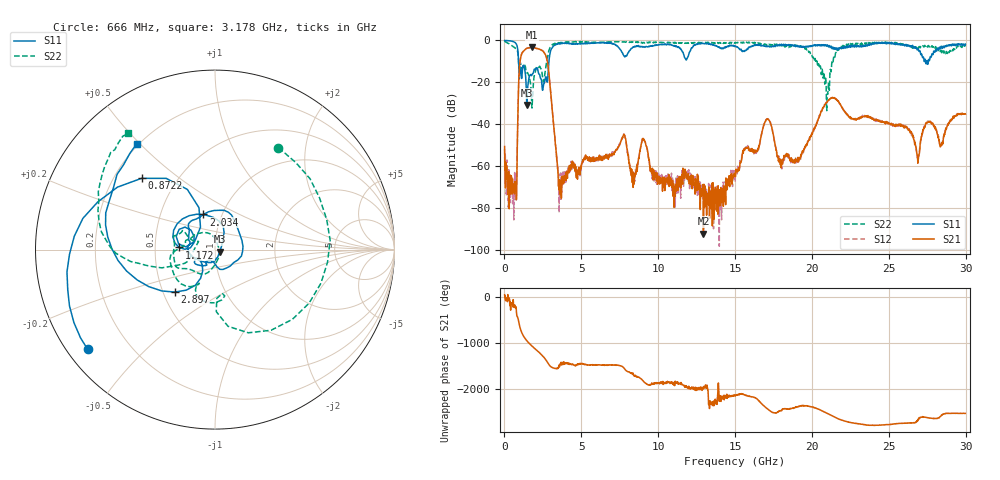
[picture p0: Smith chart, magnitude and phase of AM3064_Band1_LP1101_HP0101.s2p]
# Hz S DB R 50.0
!freq dBS11 angS11 dBS21 angS21 dBS12 angS12 dBS22 angS22
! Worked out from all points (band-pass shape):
!   1600 points, 10 MHz to 29.98 GHz, reference 50 ohm
!   highest |S21| = -3.36 dB at 1.791 GHz (marker M1); lowest = -92.1 dB at 12.94 GHz (marker M2)
!   |S21| within 3 dB of the highest: 1.125 GHz to 2.63 GHz (1.505 GHz wide, 80.2 % of centre)
!   lowest |S11| = -30.8 dB at 1.453 GHz (marker M3), VSWR 1.06, Z = 52.7 - j1.23 ohm
!   |S11| at or under -10 dB: 917.1 MHz to 2.893 GHz (1.976 GHz wide, 104 % of centre); 27.39429 GHz to 27.45839 GHz (64.1 MHz wide, 0.234 % of centre); 27.48843 GHz to 27.56216 GHz (73.73 MHz wide, 0.268 % of centre)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
!   |S22| runs from -33.5 to -0.3 dB; largest |S21 - S12| = 0.0091
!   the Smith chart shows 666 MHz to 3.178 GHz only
!   S11 on the Smith chart (normalised r, x): 666 MHz: 0.06, -0.34; 872.2 MHz: 0.31, +0.37; 1.172 GHz: 0.67, +0.02; 2.034 GHz: 0.82, +0.33; 2.897 GHz: 0.57, -0.30; 3.178 GHz: 0.19, +0.49
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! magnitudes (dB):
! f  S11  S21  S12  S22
! 10 MHz  0.0  -50.6  -51.7  -0.3
! 666 MHz  -0.9  -69.7  -63.0  -3.5
! 872.2 MHz  -4.9  -36.1  -36.2  -6.0
! 1.172 GHz  -14.0  -5.7  -5.6  -12.7
! 1.453 GHz  -30.8  -3.8  -3.7  -15.5
! 1.791 GHz  -16.3  -3.4  -3.3  -32.2
! 2.034 GHz  -13.7  -3.7  -3.7  -14.0
! 2.897 GHz  -9.7  -16.1  -16.0  -4.7
! 3.178 GHz  -2.7  -38.6  -38.6  -1.8
! 3.646 GHz  -1.5  -71.2  -63.2  -1.0
! 5.015 GHz  -1.6  -58.8  -59.2  -0.6
! 7.732 GHz  -6.9  -45.2  -45.1  -0.7
! 10 GHz  -2.1  -65.6  -64.1  -0.9
! 12.94 GHz  -1.4  -92.1  -73.6  -1.0
! 15 GHz  -2.8  -63.4  -67.4  -1.3
! 17.07 GHz  -2.7  -37.4  -37.5  -2.0
! 17.97 GHz  -2.4  -56.8  -56.7  -2.1
! 19.99 GHz  -2.9  -44.8  -44.6  -6.9
! 20.98 GHz  -2.2  -29.4  -29.1  -26.3
! 25 GHz  -1.0  -39.8  -39.1  -1.2
! 26.89 GHz  -4.0  -58.6  -56.6  -3.2
! 29.98 GHz  -1.8  -35.1  -35.1  -2.9
